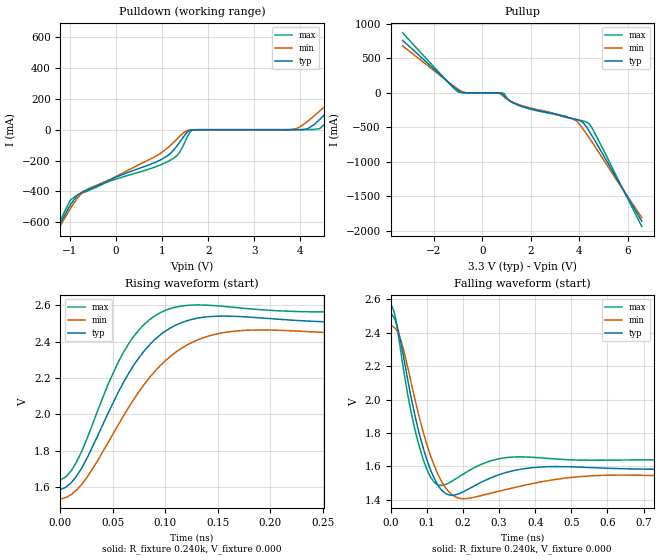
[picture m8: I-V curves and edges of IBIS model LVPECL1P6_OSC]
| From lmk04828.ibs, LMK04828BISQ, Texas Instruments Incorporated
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|   Model LVPECL1P6V
[Model]   LVPECL1P6_OSC
Model_type   Output
Polarity   Non-Inverting
Vmeas = 2.05
Vref = 1.99
Cref = 0pF
Rref = 240
|   typ   min   max
|   (nom PVT)   (fast PVT)   (slow PVT)
C_comp   0.2109p   0.1807p   0.2310p
|C_comp (Low state)   0.2109p   0.1807p   0.2310p
|C_comp (High state)   0.9933p   0.9197p   1.0724p
[Voltage Range]   3.3   3.15   3.45
[Temperature Range]   45   125   -40
[Pullup Reference]   3.3   3.15   3.45
[Pulldown Reference]   0   0   0
[Power Clamp Reference]   3.3   3.15   3.45
[GND Clamp Reference]   0   0   0
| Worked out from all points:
|   slope of the pulldown table from 0 to 0.495 V, typ, clamps not added: 8.73 ohm
|   falling waveform, R_fixture 0.240k, V_fixture 0.000: 20-80 % time 52.7ps typ, 62.3ps min, 45.2ps max; typ from 2.51 V to 1.58 V
|   rising waveform, R_fixture 0.240k, V_fixture 0.000: 20-80 % time 50ps typ, 61ps min, 41.8ps max; typ from 1.58 V to 2.51 V
[Pulldown]
|   Voltage   I(typ)   I(min)   I(max)
-3.3V     -1.869A    -1.737A    -2.051A
-1.29V    -659.3mA   -667.3mA   -647.5mA
-1.003V   -497mA     -520.8mA   -467.3mA
-825mV    -422.7mA   -440mA     -420.4mA
1.175V    -155.7mA   -103.7mA   -198.5mA
1.373V    -85.35mA   -46.2mA    -151.1mA
1.66V     -569.6uA   -270.8uA   -2.008mA
3.887V    106.5uA    6.161mA    2.469uA
4.155V    6.485mA    54.36mA    475.7uA
4.412V    65.2mA     120mA      6.277mA
5.145V    293.7mA    319.5mA    257.9mA
6.59V     761.2mA    723.2mA    811.3mA
[Pullup]
|   Voltage   I(typ)   I(min)   I(max)
-3.3V     764.4mA    683.9mA    873mA
-983.4mV  30.09mA    49.29mA    9.236mA
-686.4mV  508.5uA    3.353mA    377.6uA
561mV     -3.199uA   -263.1uA   -15.17nA
848.1mV   -23.43mA   -44.45mA   -1.6mA
1.115V    -113.4mA   -110mA     -110.4mA
1.531V    -182.7mA   -172.9mA   -185.6mA
3.739V    -374.5mA   -381.3mA   -374.9mA
4.125V    -421.7mA   -506.1mA   -405.1mA
4.392V    -544.4mA   -641.7mA   -441.8mA
4.986V    -896.2mA   -959.4mA   -816.1mA
6.59V     -1.865A    -1.813A    -1.943A
[Ramp]
R_load = 240
|   typ   min   max
dV/dt_r   0.548292/4.99905e-11   0.541543/6.09757e-11   0.55397/4.17605e-11
dV/dt_f   0.548346/5.2725e-11   0.5416/6.22718e-11   0.553999/4.51898e-11
[Falling Waveform]
R_fixture = 0.240k
V_fixture = 0.000
V_fixture_min = 0.000
V_fixture_max = 0.000
C_fixture = 0.000
|  time   V(typ)   V(min)   V(max)
0s        2.507V     2.437V     2.565V
14.04ps   2.466V     2.422V     2.482V
29.04ps   2.332V     2.348V     2.275V
74.04ps   1.842V     1.939V     1.762V
104ps     1.617V     1.705V     1.564V
134ps     1.478V     1.539V     1.488V
194ps     1.441V     1.408V     1.545V
344ps     1.577V     1.474V     1.657V
599ps     1.589V     1.547V     1.637V
1.869ns   1.584V     1.535V     1.639V
[Rising Waveform]
R_fixture = 0.240k
V_fixture = 0.000
V_fixture_min = 0.000
V_fixture_max = 0.000
C_fixture = 0.000
|  time   V(typ)   V(min)   V(max)
0s        1.584V     1.535V     1.639V
10.37ps   1.624V     1.558V     1.69V
20.37ps   1.705V     1.615V     1.797V
45.37ps   2.006V     1.844V     2.165V
70.37ps   2.275V     2.087V     2.433V
90.37ps   2.414V     2.239V     2.544V
120.4ps   2.515V     2.381V     2.6V
150.4ps   2.541V     2.445V     2.597V
190.4ps   2.531V     2.465V     2.577V
1.885ns   2.507V     2.438V     2.565V
